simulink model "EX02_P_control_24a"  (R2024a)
settings: Solver=ode45  StartTime=0.0  StopTime=50  MaxStep=1e-3  RelTol=1e-3  EnableMultiTasking=on

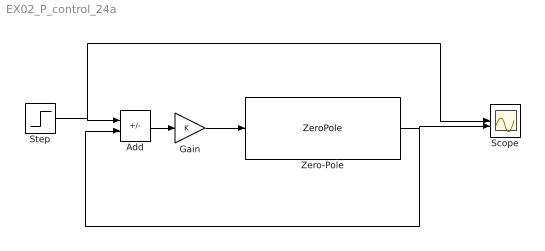
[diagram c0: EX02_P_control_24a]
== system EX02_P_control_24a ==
  Add : Sum  Inputs=+-
  Gain : Gain
  Scope : Scope  NumInputPorts=2
  Step : Step  Time=0  SampleTime=0
  Zero-Pole : ZeroPole  Zeros=[]  Poles=[0 -1 -2]  Gain=1
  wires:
  Zero-Pole/1 -> Scope/2, Add/2
  Gain/1 -> Zero-Pole/1
  Add/1 -> Gain/1
  Step/1 -> Scope/1, Add/1
